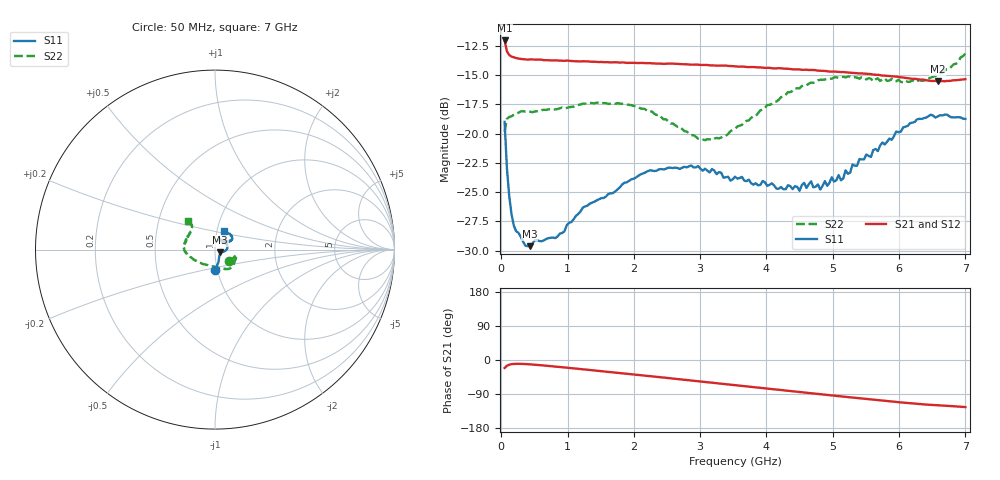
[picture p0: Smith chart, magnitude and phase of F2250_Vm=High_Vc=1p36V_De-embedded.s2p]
! Integrated Device Technology
! Corporate Headquarters
! 6024 Silver Creek Valley Road
! San Jose, CA 95138  USA
! Phone:  1-408-284-8200
! Toll Free:  1-800-223-1366
! Webpage:  http://www.idt.com/
! Timing and RF Division
! 515 Groton Road, Suite 102
! Westford, MA 01886-6024
! Device:  F2250
! Description: Voltage Variable RF Attenuator
! Frequency:  50.0 -  6000.00 MHz
! Package:  3x3 mm Thin QFN Plastic Package: 16 pin
! Ports:  2 RF, 3 DC
!  Pin  1  = GND
!  Pin  2  = NC
!  Pin  3  = RF1  = Port 1
!  Pin  4  = NC
!  Pin  5  = GND
!  Pin  6  = GND
!  Pin  7  = GND
!  Pin  8  = GND
!  Pin  9  = NC
!  Pin 10  = RF2  = Port 2
!  Pin 11  = NC
!  Pin 12  = GND
!  Pin 13  = GND
!  Pin 14  = VCNTRL
!  Pin 15  = VDD
!  Pin 16  = VMODE
! Vcntrl:  1.360 Volts
! Vmode:  +3.300 Volts
! Vdd:  +3.30  Volts
! Current:  1.331 mA
! Data:  The device was measured on a the F2250 evaluation board which has
!  individual transmission lines to the RF pins.  Data was collected
!  using a calibrated network analyzer.  The evaluation board was
!  de-embedded using a TRL calibration technique.
!  The reference plane is the edge of the package pin.
! Misc:  SN 10
!  Action Tracker AT0258
! Date Measured:  2014-11-26
! Date:  2015-10-15  MJV
! Note:
!  Integrated Device Technology supplies this data as a sample of measured
!  data at the package pin for this product.  Your particular data for this
!  product may vary.
!  Data was taken at 25 degrees C.
!  Integrated Device Technology reserves the right to change this data at anytime.
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# GHz S dB R 50
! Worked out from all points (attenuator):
!   201 points, 50 MHz to 7 GHz, reference 50 ohm
!   highest |S21| = -12.04 dB at 50 MHz (marker M1); lowest = -15.5 dB at 6.583 GHz (marker M2)
!   lowest |S11| = -29.6 dB at 432.2 MHz (marker M3), VSWR 1.07, Z = 53 - j1.61 ohm
!   |S11| at or under -10 dB: start of sweep to end of sweep
!   |S22| runs from -20.6 to -13.2 dB; largest |S21 - S12| = 0.00083
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0.05  -19.00 -89.1  -12.04 -21.0  -12.03 -20.9  -19.84 -39.9
0.08475  -22.95 -73.9  -12.96 -15.2  -12.96 -15.2  -18.74 -21.0
0.1195  -25.34 -65.7  -13.28 -12.4  -13.30 -12.4  -18.58 -15.5
0.189  -27.87 -50.8  -13.48 -10.4  -13.49 -10.4  -18.40 -13.7
0.43225  -29.63 -27.4  -13.65 -11.4  -13.65 -11.4  -18.13 -16.4
0.8145  -28.94 -16.8  -13.75 -17.3  -13.74 -17.3  -17.94 -28.5
1.2315  -26.32 -14.9  -13.82 -24.6  -13.82 -24.6  -17.43 -39.7
1.857  -24.20 -3.3  -13.92 -35.7  -13.93 -35.7  -17.46 -52.3
2.37825  -23.05 9.3  -14.01 -45.1  -14.02 -45.1  -18.39 -64.4
3.07325  -23.00 30.7  -14.13 -58.0  -14.11 -58.0  -20.56 -99.4
3.525  -23.68 46.9  -14.25 -66.4  -14.26 -66.4  -19.59 -130.7
4.1505  -24.71 64.1  -14.42 -77.9  -14.41 -78.0  -17.25 -160.0
4.498  -24.89 61.7  -14.52 -84.4  -14.54 -84.4  -16.14 -170.6
4.67175  -24.08 60.9  -14.56 -87.7  -14.57 -87.7  -15.64 -174.4
4.7065  -24.59 61.5  -14.56 -88.3  -14.58 -88.3  -15.66 -175.0
5.08875  -23.55 48.5  -14.73 -95.3  -14.72 -95.4  -15.24 176.7
5.1235  -23.99 48.7  -14.74 -96.0  -14.73 -96.0  -15.17 175.7
5.193  -23.14 43.8  -14.76 -97.2  -14.77 -97.3  -15.19 174.6
5.85325  -20.43 30.4  -15.08 -109.0  -15.08 -109.1  -15.46 157.7
6.27025  -18.79 32.7  -15.34 -115.8  -15.35 -115.8  -15.56 144.5
6.583  -18.53 40.7  -15.54 -119.6  -15.55 -119.7  -14.94 135.6
7  -18.74 65.3  -15.35 -124.3  -15.34 -124.5  -13.16 133.9
